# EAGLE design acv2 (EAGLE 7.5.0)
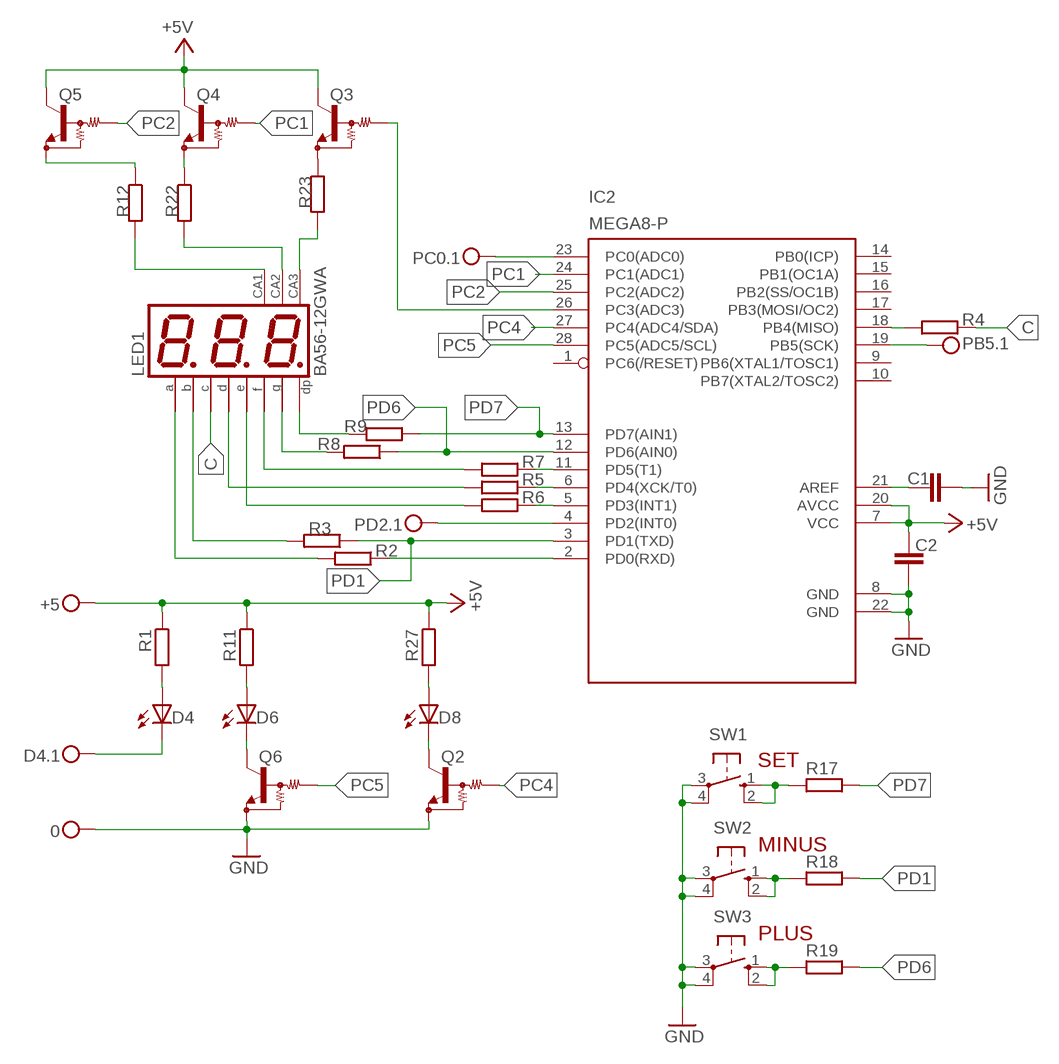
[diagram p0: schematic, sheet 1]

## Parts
0  CONNWIRE  [CONNWIRE]
+5  CONNWIRE  [CONNWIRE]
C1  C-EUC1206  [C1206]
C2  C-EUC1206  [C1206]
D4  LED3MM  [LED3MM]
D4.1  CONNWIRE  [CONNWIRE]
D6  LED3MM  [LED3MM]
D8  LED3MM  [LED3MM]
IC2  MEGA8-P  [DIL28-3]
LED1  BA56-12GWA  [BX56-12]
PB5.1  CONNWIRE  [CONNWIRE]
PC0.1  CONNWIRE  [CONNWIRE]
PD2.1  CONNWIRE  [CONNWIRE]
Q2  MUN2211T1-NPN_DRIVER-SC59-BEC  [SC59-BEC]
Q3  MUN2211T1-NPN_DRIVER-SC59-BEC  [SC59-BEC]
Q4  MUN2211T1-NPN_DRIVER-SC59-BEC  [SC59-BEC]
Q5  MUN2211T1-NPN_DRIVER-SC59-BEC  [SC59-BEC]
Q6  MUN2211T1-NPN_DRIVER-SC59-BEC  [SC59-BEC]
R1  R-EU_M1206  [M1206]
R2  R-EU_M1206  [M1206]
R3  R-EU_M1206  [M1206]
R4  R-EU_M1206  [M1206]
R5  R-EU_M1206  [M1206]
R6  R-EU_M1206  [M1206]
R7  R-EU_M1206  [M1206]
R8  R-EU_M1206  [M1206]
R9  R-EU_M1206  [M1206]
R11  R-EU_M1206  [M1206]
R12  R-EU_M1206  [M1206]
R17  R-EU_M1206  [M1206]
R18  R-EU_M1206  [M1206]
R19  R-EU_M1206  [M1206]
R22  R-EU_M1206  [M1206]
R23  R-EU_M1206  [M1206]
R27  R-EU_M1206  [M1206]
SW1  10-XX  [B3F-10XX]
SW2  10-XX  [B3F-10XX]
SW3  10-XX  [B3F-10XX]

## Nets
+5V: +5.P$1 C2.1 IC2.7(VCC) IC2.20(AVCC) Q3.C Q4.C Q5.C R1.1 R11.1 R27.1
C: LED1.4(C) R4.1
GND: 0.P$1 C1.1 C2.2 IC2.8(GND) IC2.22(GND) Q2.E Q6.E SW1.3(P) SW1.4(P1) SW2.3(P) SW2.4(P1) SW3.3(P) SW3.4(P1)
N$1: D8.A R27.2
N$2: D8.K(C) Q2.C
N$3: D6.A R11.2
N$4: D6.K(C) Q6.C
N$5: D4.A R1.2
N$6: IC2.4(PD2(INT0)) PD2.1.P$1
N$7: D4.1.P$1 D4.K(C)
N$8: R17.2 SW1.1(S) SW1.2(S1)
N$9: R18.2 SW2.1(S) SW2.2(S1)
N$10: R19.2 SW3.1(S) SW3.2(S1)
N$11: LED1.8(CA) R23.2
N$13: IC2.2(PD0(RXD)) R2.1
N$16: IC2.11(PD5(T1)) R7.1
N$17: IC2.6(PD4(XCK/T0)) R5.1
N$18: IC2.5(PD3(INT1)) R6.1
N$19: LED1.7(B) R3.2
N$20: LED1.11(A) R2.2
N$21: LED1.3(DP) R9.2
N$22: LED1.5(G) R8.2
N$23: LED1.10(F) R7.2
N$24: Q5.E R12.1
N$26: IC2.23(PC0(ADC0)) PC0.1.P$1
N$27: IC2.18(PB4(MISO)) R4.2
N$32: IC2.19(PB5(SCK)) PB5.1.P$1
N$33: LED1.2(D) R5.2
N$34: LED1.1(E) R6.2
N$35: LED1.12(CA) R12.2
N$36: LED1.9(CA) R22.2
N$37: Q4.E R22.1
N$38: Q3.E R23.1
N$39: C1.2 IC2.21(AREF)
PC1: IC2.24(PC1(ADC1)) Q4.B
PC2: IC2.25(PC2(ADC2)) Q5.B
PC3: IC2.26(PC3(ADC3)) Q3.B
PC4: IC2.27(PC4(ADC4/SDA)) Q2.B
PC5: IC2.28(PC5(ADC5/SCL)) Q6.B
PD1: IC2.3(PD1(TXD)) R3.1 R18.1
PD6: IC2.12(PD6(AIN0)) R8.1 R19.1
PD7: IC2.13(PD7(AIN1)) R9.1 R17.1
Unconnected: IC2.1(PC6(/RESET)) IC2.9(PB6(XTAL1/TOSC1)) IC2.10(PB7(XTAL2/TOSC2)) IC2.14(PB0(ICP)) IC2.15(PB1(OC1A)) IC2.16(PB2(SS/OC1B)) IC2.17(PB3(MOSI/OC2))

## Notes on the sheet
- SET
- MINUS
- PLUS

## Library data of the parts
0 +5 D4.1 PB5.1 PC0.1 PD2.1 = connholes:CONNWIRE
C1 C2 = rcl:C-EU: CAPACITOR, European symbol
D4 D6 D8 = led:LED: LED
IC2 = atmel:MEGA8-P: MICROCONTROLLER 8 Kbytes FLASH, 1 kbytes SRAM, 512 bytes EEPROM, USART, 4-channel 10 bit ADC, 2-channel 8 bit ADC Pin compatible with Atmega48, ATMega88, ATMega168 Source: avr.lbr; OC_FARNELL: unknown; OC_NEWARK: unknown
LED1 = display-kingbright:B?56-12*WA: 14.22mm (0.56INCH) THREE DIGIT NUMERIC DISPLAY Source: http://www.kingbright.com .. BA56-11EWA(Ver1189474895.pdf; OC_FARNELL: unknown; OC_NEWARK: unknown
Q2-Q6 = transistor:*-NPN_DRIVER-: NPN Bias Resistor Transistor
R1-R9 R11 R12 R17-R19 R22 R23 R27 = resistor:R-EU_: RESISTOR, European symbol
SW1-SW3 = switch-omron:10-XX: OMRON SWITCH; MPN: B3F-1000; OC_FARNELL: 176432; OC_NEWARK: 36M3542

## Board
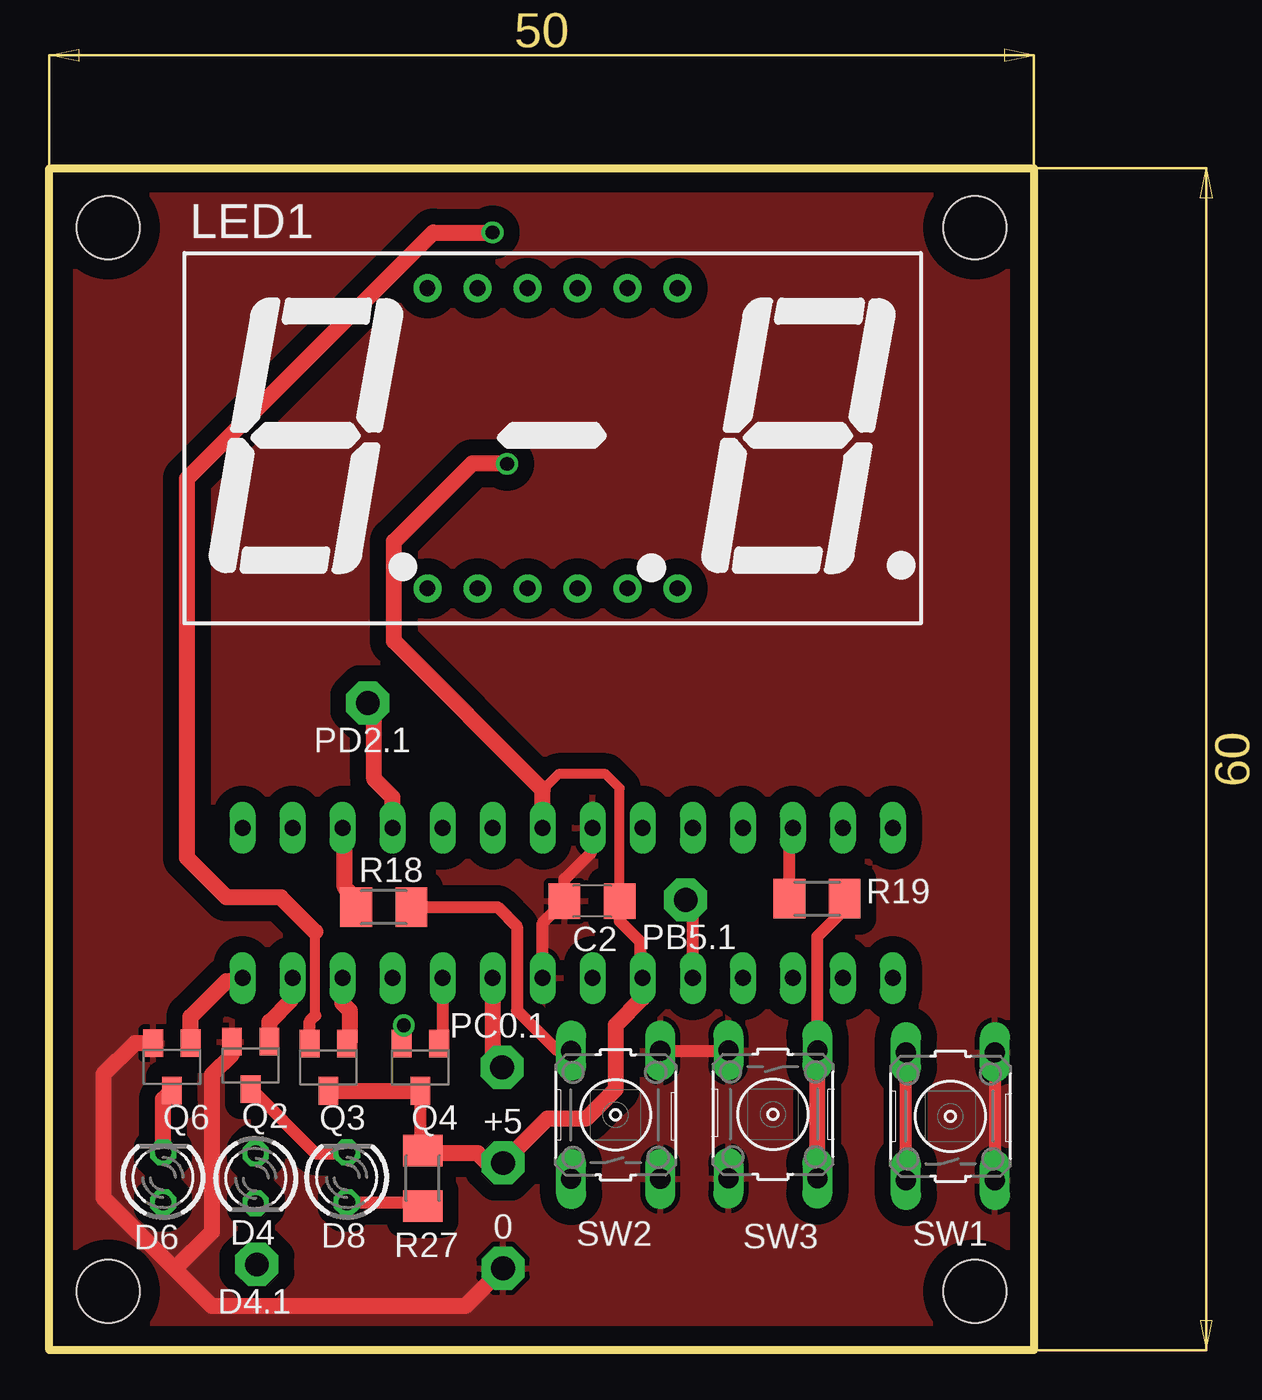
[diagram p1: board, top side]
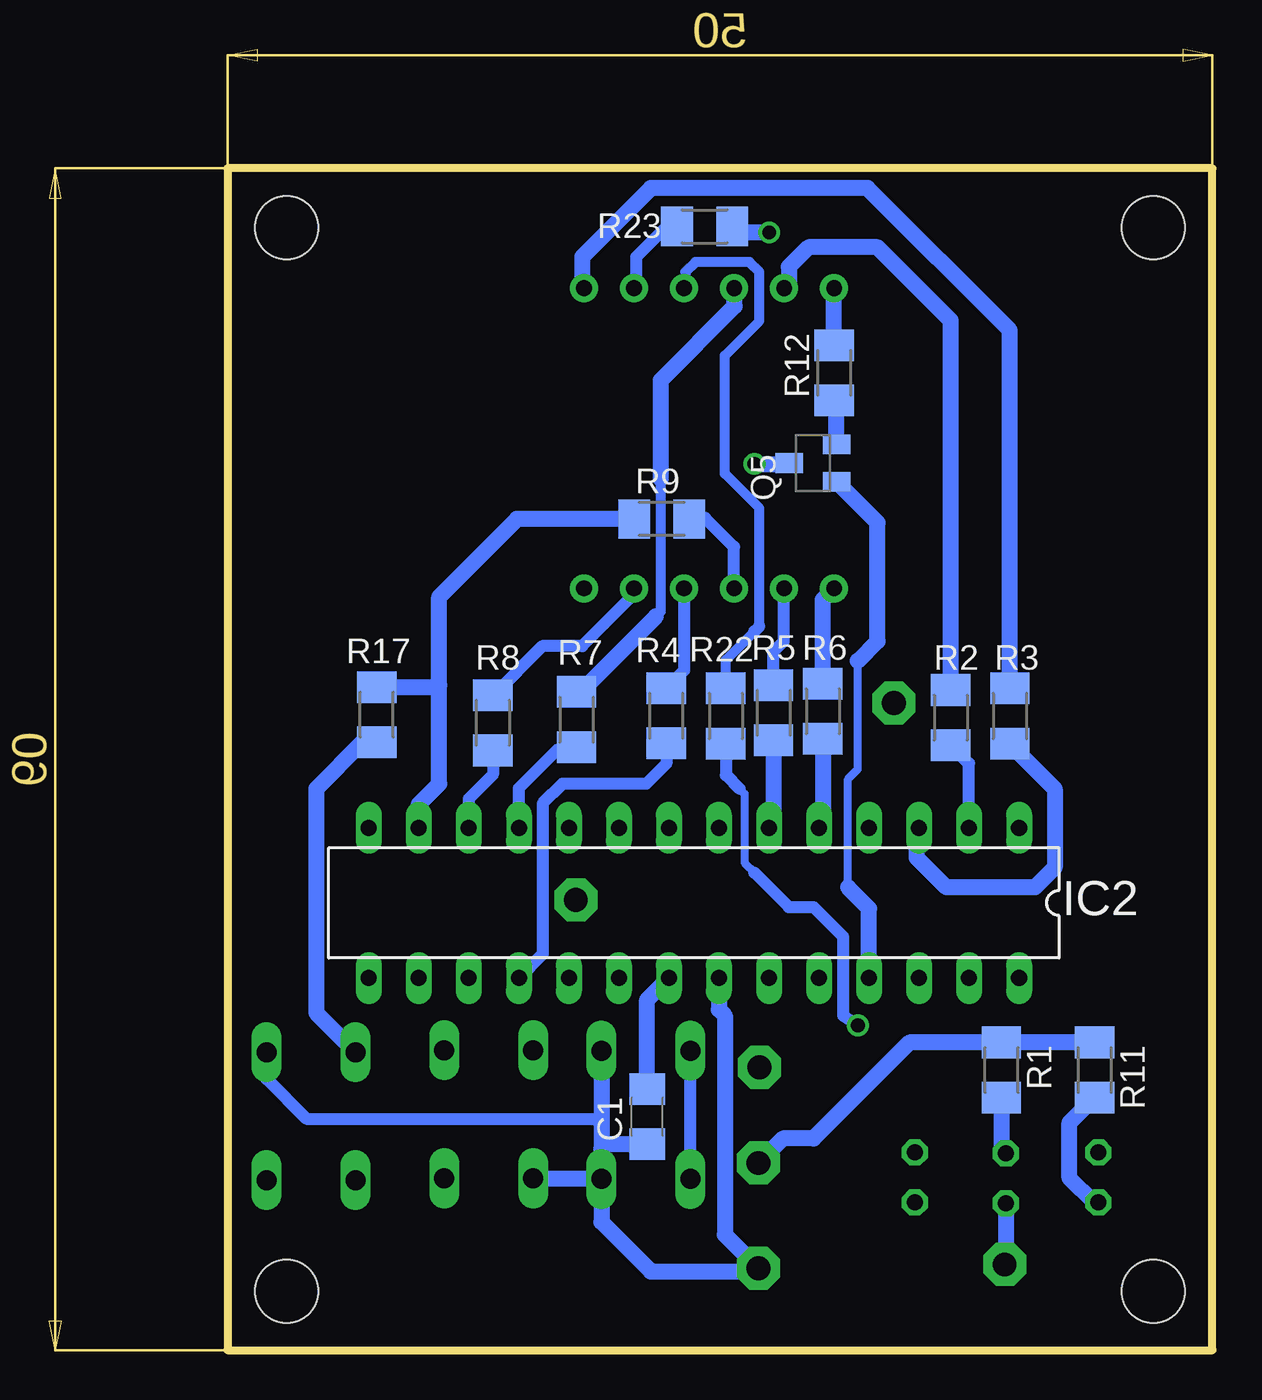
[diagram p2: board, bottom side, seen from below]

Size 59.05 x 66.05 mm. Coordinates in mm from the lower left corner, seen from the top.
Outline: 0,0 0,60 50,60 50,0 0,0
Copper layers (1*16): Top 0.035mm / dielectric 1.5mm / Bottom 0.035mm
Design rules "default": minimum track width 10mil, minimum drill 24mil, track to track 8mil, track to pad 8mil, pad to pad 8mil, via to via 8mil, smd to smd 8mil, copper to edge 40mil, drill to drill 8mil, minimum pad ring 10mil, minimum via ring 8mil, stop-mask expansion 4mil, vias tented up to drill 0mil, thermal gap 10mil
Holes 3.2 mm at 3,57 47,57 3,3 47,3

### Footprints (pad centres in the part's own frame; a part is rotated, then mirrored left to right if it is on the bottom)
CONNWIRE = drill 1.2 pad 2.184 octagon: P$1 0,0
C1206 = smd 1.6 x 1.8: 1 -1.4,0; 2 1.4,0
LED3MM = drill 0.813 octagon: A -1.27,0; K 1.27,0
DIL28-3 = drill 0.813 long: 1 -16.51,-3.81; 2 -13.97,-3.81; 3 -11.43,-3.81; 4 -8.89,-3.81; 5 -6.35,-3.81; 6 -3.81,-3.81; 7 -1.27,-3.81; 8 1.27,-3.81; 9 3.81,-3.81; 10 6.35,-3.81; 11 8.89,-3.81; 12 11.43,-3.81; 13 13.97,-3.81; 14 16.51,-3.81; 15 16.51,3.81; 16 13.97,3.81; 17 11.43,3.81; 18 8.89,3.81; 19 6.35,3.81; 20 3.81,3.81; 21 1.27,3.81; 22 -1.27,3.81; 23 -3.81,3.81; 24 -6.35,3.81; 25 -8.89,3.81; 26 -11.43,3.81; 27 -13.97,3.81; 28 -16.51,3.81
BX56-12 = drill 0.8 pad 1.422: 1 -6.35,-7.62; 2 -3.81,-7.62; 3 -1.27,-7.62; 4 1.27,-7.62; 5 3.81,-7.62; 6 6.35,-7.62; 7 6.35,7.62; 8 3.81,7.62; 9 1.27,7.62; 10 -1.27,7.62; 11 -3.81,7.62; 12 -6.35,7.62
SC59-BEC = smd 1 x 1.4: B -0.95,-1.2; C 0,1.2; E 0.95,-1.2
M1206 = smd 1.6 x 2: 1 -1.4,0; 2 1.4,0
B3F-10XX = drill 1.016 long: 1 -3.251,2.261; 2 3.251,2.261; 3 -3.251,-2.261; 4 3.251,-2.261

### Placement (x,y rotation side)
0  23.04,4.16 0 top
+5  23.04,9.51 0 top
C1  28.7,11.86 90 bottom
C2  27.56,22.8 180 top
D4  10.48,8.73 270 top
D4.1  10.54,4.36 0 top
D6  5.78,8.77 90 top
D8  15.11,8.77 90 top
IC2  26.32,22.71 180 bottom
LED1  25.55,46.3 0 top
PB5.1  32.31,22.86 0 top
PC0.1  22.99,14.36 0 top
PD2.1  16.17,32.86 0 top
Q2  10.23,14.46 180 top
Q3  14.17,14.37 180 top
Q4  18.84,14.37 180 top
Q5  20.28,45.04 90 bottom
Q6  6.23,14.39 180 top
R1  10.71,14.23 270 bottom
R2  13.28,32.12 90 bottom
R3  10.28,32.2 90 bottom
R4  27.72,32.22 270 bottom
R5  22.28,32.36 90 bottom
R6  19.78,32.44 90 bottom
R7  32.28,32.02 90 bottom
R8  36.53,31.85 90 bottom
R9  27.96,42.2 0 bottom
R11  5.97,14.23 270 bottom
R12  19.2,49.62 90 bottom
R17  42.42,32.27 270 bottom
R18  16.98,22.5 0 top
R19  38.98,22.92 0 top
R22  24.7,32.2 90 bottom
R23  25.78,57.05 180 bottom
R27  18.96,8.73 270 top
SW1  45.76,11.88 90 top
SW2  28.76,11.95 90 top
SW3  36.74,11.98 270 top

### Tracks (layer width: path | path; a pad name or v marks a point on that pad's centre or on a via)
+5V  (via drill 0.7)
  Top 0.5: C2.1 28.96,28.54 28.25,29.25 25.85,29.25 25.05,28.45
  Top 0.61: Q4.C 18.84,10.25 R27.1 | C2.1 28.96,21.79 30,20.75 30,19.03 IC2.20
  Top 0.813: R27.1 19.09,10 21.75,10 22.24,9.51 +5.P$1 25.28,11.75 27.25,11.75 28.75,13.25 28.75,16.5 30.13,17.88 IC2.20 | Q3.C Q4.C | IC2.7 25.05,28.45 17.5,36 17.5,41.06 Q5.C 23.21,45.04 v23.25,45
  Bottom 0.813: R11.1 R1.1 15.37,15.63 20.25,10.75 21.8,10.75 +5.P$1 | v23.25,45 21.52,45 Q5.C
C
  Bottom 0.61: LED1.4 26.82,34.52 R4.1
GND
  Top 0.61: IC2.22 25.05,21.69 C2.2 26.16,23.91 27.5,25.25 27.5,26.43 IC2.8 | SW2.4 34.45,15.2 SW3.3 | SW1.4 SW1.3
  Top 0.813: Q6.E 4.34,15.59 2.75,14 2.75,7.75 6.38,4.12 | 6.38,4.12 8.25,2.25 21.13,2.25 0.P$1 | Q2.E 9.28,15.03 8.25,14 8.25,6 6.38,4.12
  Bottom 0.61: SW1.4 48.02,13.77 46,11.75 31.27,11.75 31.02,11.5
  Bottom 0.813: SW2.4 31.02,11.5 31.02,10.25 | 31.02,10.25 SW2.3 | SW2.3 31.02,6.52 28.5,4 23.2,4 0.P$1 24.75,5.87 24.75,17 25.05,17.3 IC2.22 | C1.1 30.81,10.46 31.02,10.25 | SW3.4 31.05,8.73 SW2.3
  pour Top (isolate 0.813): 0.5,59.5 49.5,59.5 49.5,0.5 0.5,0.5
N$1
  Top 0.61: D8.A 18.79,7.5 R27.2
N$2
  Top 0.61: Q2.C 13.5,10 15.07,10 D8.K
N$3
  Bottom 0.813: D6.A 6,7.5 7.25,8.75 7.25,11.55 R11.2
N$4
  Top 0.813: D6.K 5.78,12.74 Q6.C
N$5
  Bottom 0.813: R1.2 10.71,10.23 D4.A
N$6
  Top 0.813: IC2.4 17.43,28.07 16.5,29 16.5,32.69 PD2.1.P$1
N$7
  Bottom 0.813: D4.K 10.48,4.42 D4.1.P$1
N$8
  Top 0.61: SW1.1 SW1.2
  Bottom 0.813: R17.2 43.13,30.87 45.5,28.5 45.5,17.13 SW1.2
N$9
  Top 0.61: R18.2 22.75,22.5 23.75,21.5 23.75,17.25 25.75,15.25 26.45,15.25 SW2.2
  Bottom 0.61: SW2.1 SW2.2
N$10
  Top 0.61: SW3.1 39,21 40.25,22.25 40.25,22.79 R19.2
  Top 0.813: SW3.2 SW3.1
N$11
  Bottom 0.61: R23.2 27.7,57.05 29.25,55.5 29.25,54.03 LED1.8
N$13
  Bottom 0.61: IC2.2 12.35,29.79 R2.1
N$16
  Bottom 0.61: IC2.11 35.21,28.54 33.25,30.5 32.4,30.5 R7.1
N$17
  Bottom 0.813: R5.1 22.28,26.75 IC2.6
N$18
  Bottom 0.813: R6.1 19.78,26.71 IC2.5
N$19
  Bottom 0.813: R3.2 10.28,51.78 17.5,59 28.5,59 32,55.5 32,54.02 LED1.7
N$20
  Bottom 0.813: R2.2 13.28,52.28 17,56 20.5,56 21.5,55 21.5,54.16 LED1.11
N$21
  Bottom 0.61: LED1.3 24.28,40.78 25.75,42.25 26.51,42.25 R9.2
N$22
  Bottom 0.61: LED1.5 29.36,38.39 32,35.75 34.03,35.75 R8.2
N$23
  Bottom 0.5: 28.25,37.25 28,37.5 28,44.25
  Bottom 0.813: R7.2 32.08,33.42 28.25,37.25 | 28,44.25 28,49.25 24.25,53 24.25,53.89 LED1.10
N$24
  Bottom 0.813: Q5.E 19.08,48.1 R12.1
N$26
  Top 0.813: IC2.23 22.51,14.84 PC0.1.P$1
N$27
  Bottom 0.61: R4.2 27.72,29.78 28.75,28.75 33,28.75 34,27.75 34,20.11 IC2.18
N$32
  Top 0.61: IC2.19 32.67,22.5 PB5.1.P$1
N$33
  Bottom 0.61: R5.2 22.28,35.47 21.75,36 LED1.2
N$34
  Bottom 0.813: R6.2 19.78,38.1 LED1.1
N$35
  Bottom 0.813: R12.2 LED1.12
N$36
  Bottom 0.5: R22.2 24.7,35.05 23.25,36.5 | 23,36.75 23,42.75 24.75,44.5 24.75,50.5 23,52.25 23,54.75 23.5,55.25 26.25,55.25 26.75,54.75 26.75,53.99 LED1.9
  Bottom 0.61: 23.25,36.5 23,36.75
N$37  (via drill 0.7)
  Top 0.61: v18,16.5 18,15.93 Q4.E
  Bottom 0.406: 24,28.5 23.75,28.25 23.75,24.75 23.25,24.25
  Bottom 0.61: R22.1 24.7,29.2 24,28.5 | 23.25,24.25 21.5,22.5 20.25,22.5 18.75,21 18.75,17 v18,16.5
N$38  (via drill 0.7)
  Top 0.5: 13.5,17 13.5,21.25
  Top 0.61: Q3.E 13.22,16.72 13.5,17
  Top 0.813: v22.5,56.75 19.5,56.75 7,44.25 7,25 9,23 11.75,23 13.5,21.25
  Bottom 0.813: v22.5,56.75 24.33,56.75 R23.1
N$39
  Bottom 0.813: C1.2 28.7,17.79 IC2.21
PC1
  Top 0.61: IC2.24 19.97,15.75 Q4.B
PC2
  Bottom 0.406: 18.5,23.5 18.5,29 18,29.5 18,35
  Bottom 0.813: IC2.25 17.43,22.43 18.5,23.5 | 18,35 17,36 17,42.01 Q5.B
PC3
  Top 0.813: IC2.26 14.89,17.61 15.25,17.25 15.25,15.7 Q3.B
PC4
  Top 0.813: Q2.B 11.18,16.68 12.25,17.75 12.25,18.8 IC2.27
PC5
  Top 0.813: Q6.B 7.18,16.93 9,18.75 9.66,18.75 IC2.28
PD1
  Top 0.813: R18.1 15.58,22.92 15,23.5 15,26.41 IC2.3
  Bottom 0.813: R3.1 10.28,30.78 8,28.5 8,24.5 9,23.5 13.5,23.5 15,25 15,26.41 IC2.3
PD6
  Top 0.61: R19.1 37.58,26.35 IC2.12
  Bottom 0.61: R8.1 36.53,29.22 37.75,28 IC2.12
PD7
  Bottom 0.813: R9.1 35.3,42.2 39.25,38.25 39.25,33.75 | IC2.13 40.29,27.71 39.25,28.75 39.25,33.75 | R17.1 39.33,33.67 39.25,33.75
